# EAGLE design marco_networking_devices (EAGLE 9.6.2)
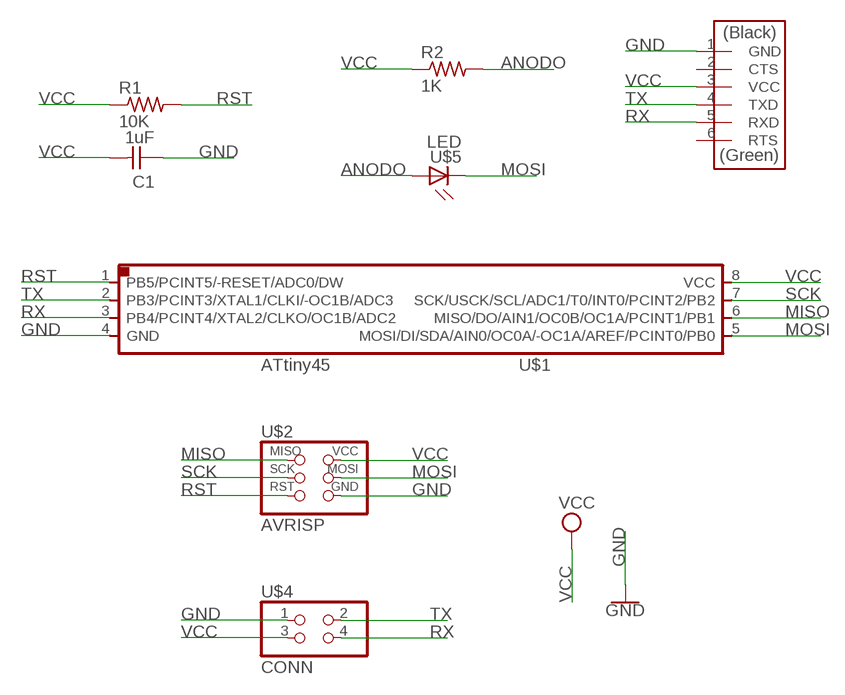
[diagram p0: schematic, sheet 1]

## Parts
C1  1uF  CAP_UNPOLARIZEDFAB  [C1206FAB]
R1  10K  R1206FAB  [R1206FAB]
R2  1K  R1206FAB  [R1206FAB]
U$1  ATTINY45  UC_ATTINY45SI  [SOIC8]
U$2  AVRISP  CONN_03X2_AVRISPSMD  [2X03SMD]
U$3  FTDI  CONN_06_FTDI-SMD-HEADER  [1X06SMD]
U$4  CONN  CONN_02X2-PINHEAD-SMD  [2X02SMD]
U$5  LED  LEDFAB1206  [LED1206FAB]

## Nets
ANODO: R2.2 U$5.1(A)
GND: C1.1 U$1.4(GND) U$2.6(GND) U$3.1(GND) U$4.1
MISO: U$1.6(MISO/DO/AIN1/OC0B/OC1A/PCINT1/PB1) U$2.1(MISO)
MOSI: U$1.5(MOSI/DI/SDA/AIN0/OC0A/-OC1A/AREF/PCINT0/PB0) U$2.4(MOSI) U$5.2(C)
RST: R1.2 U$1.1(PB5/PCINT5/-RESET/ADC0/DW) U$2.5(RST)
RX: U$1.3(PB4/PCINT4/XTAL2/CLKO/OC1B/ADC2) U$3.5(RXD) U$4.4
SCK: U$1.7(SCK/USCK/SCL/ADC1/T0/INT0/PCINT2/PB2) U$2.3(SCK)
TX: U$1.2(PB3/PCINT3/XTAL1/CLKI/-OC1B/ADC3) U$3.4(TXD) U$4.2
VCC: C1.2 R1.1 R2.1 U$1.8(VCC) U$2.2(VCC) U$3.3(VCC) U$4.3
Unconnected: U$3.2(CTS) U$3.6(RTS)

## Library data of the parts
C1 = fab:CAP_UNPOLARIZED
R1 R2 = fab:R: Resistor (US Symbol)
U$1 = fab:UC_ATTINY45
U$2 = fab:CONN_03X2_AVRISP
U$3 = fab:CONN_06_FTDI-SMD-HEADER
U$4 = fab:CONN_02X2-PINHEAD-SMD
U$5 = fab:LED: LED

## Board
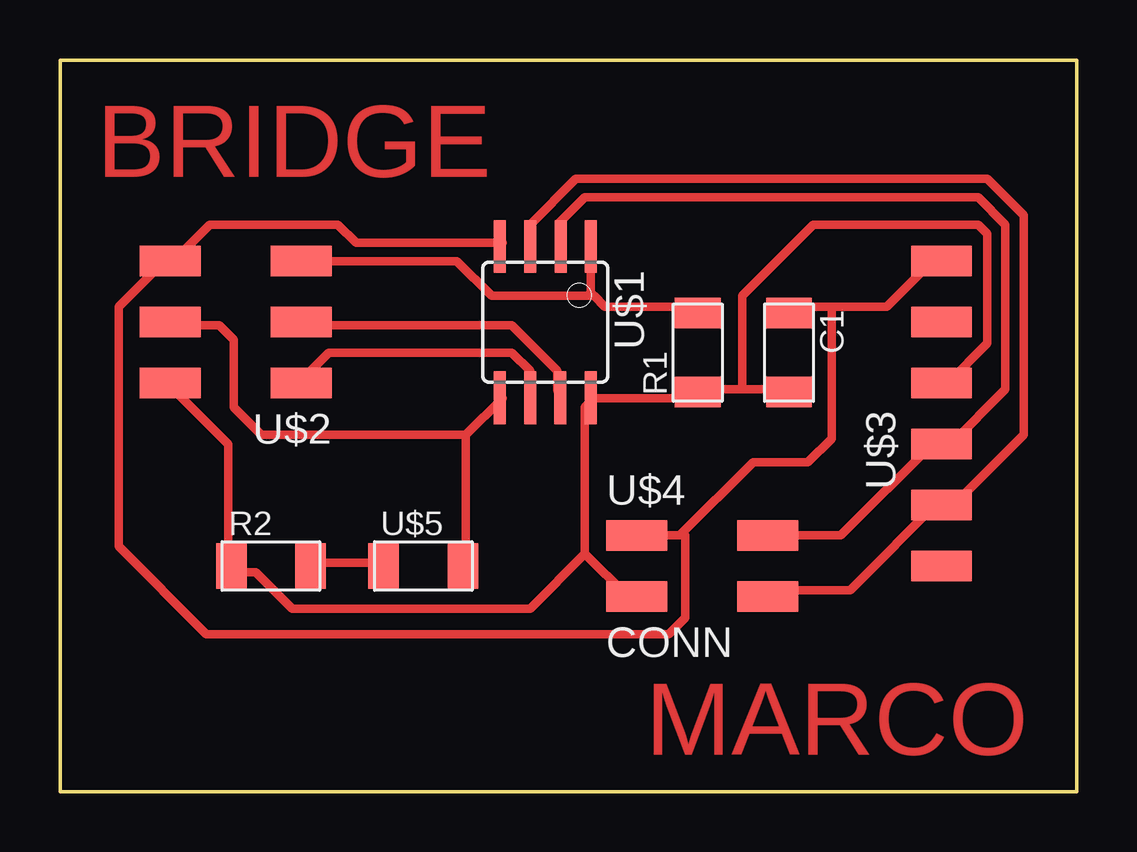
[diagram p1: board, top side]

Size 42.37 x 30.48 mm. Coordinates in mm from the lower left corner, seen from the top.
Outline: 0,30.48 42.37,30.48 42.37,0 0,0 0,30.48
Copper layers (1*16): Top 0.035mm / dielectric 1.5mm / Bottom 0.035mm
Design rules "fabcity-designrules *": minimum track width 14mil, minimum drill 32mil, track to track 16mil, track to pad 16mil, pad to pad 16mil, via to via 16mil, smd to smd 6mil, copper to edge 16mil, drill to drill 16mil, minimum pad ring 10mil, minimum via ring 8mil, stop-mask expansion 4mil, vias tented up to drill 0mil, thermal gap 16mil

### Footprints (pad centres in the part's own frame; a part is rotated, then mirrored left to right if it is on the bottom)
C1206FAB = smd 1.27 x 1.905: 1 -1.651,0; 2 1.651,0
R1206FAB = smd 1.27 x 1.905: 1 -1.651,0; 2 1.651,0
SOIC8 = smd 0.5 x 2.2: 1 -1.905,-3.154; 2 -0.645,-3.154; 3 0.625,-3.154; 4 1.895,-3.154; 5 1.905,3.154; 6 0.635,3.154; 7 -0.635,3.154; 8 -1.905,3.154
2X03SMD = smd 2.54 x 1.27: 1 -2.54,2.54; 2 2.92,2.54; 3 -2.54,0; 4 2.92,0; 5 -2.54,-2.54; 6 2.92,-2.54
1X06SMD = smd 2.54 x 1.27: 1 0,6.35; 2 0,3.81; 3 0,1.27; 4 0,-1.27; 5 0,-3.81; 6 0,-6.35
2X02SMD = smd 2.54 x 1.27: 1 -2.54,1.27; 2 2.92,1.27; 3 -2.54,-1.27; 4 2.92,-1.27
LED1206FAB = smd 1.27 x 1.905: 1 -1.651,0; 2 1.651,0

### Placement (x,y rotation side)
C1  30.38,18.29 270 top
R1  26.57,18.29 90 top
R2  8.79,9.4 0 top
U$1  20.22,19.56 180 top
U$2  7.52,19.56 180 top
U$3  36.73,15.75 0 top
U$4  26.57,9.4 0 top
U$5  15.14,9.4 0 top

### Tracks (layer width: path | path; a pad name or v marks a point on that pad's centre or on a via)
ANODO
  Top 0.356: R2.2 10.44,9.53 13.49,9.53 U$5.1
GND
  Top 0.356: U$1.4 18.44,22.86 12.34,22.86 11.58,23.62 6.25,23.62 4.72,22.1 U$2.6 4.34,22.1 2.44,20.19 2.44,10.21 6.1,6.55 25.37,6.55 26.06,7.24 26.06,10.67 25.83,10.67 | 32.16,20.19 34.44,20.19 36.35,22.1 U$3.1 | 32.16,20.19 30.63,20.19 C1.1 | 25.83,10.67 U$4.1 | 25.83,10.67 28.88,13.72 31.17,13.72 32.16,14.71 32.16,20.19
MISO
  Top 0.356: U$1.6 19.58,17.53 18.82,18.29 11.2,18.29 10.06,17.14 U$2.1
MOSI
  Top 0.356: 16.92,14.86 16.92,9.53 U$5.2 | 16.92,14.86 18.44,16.38 U$1.5 | 16.92,14.86 8.38,14.86 7.24,16 7.24,18.82 6.63,19.43 4.72,19.43 U$2.4
RST
  Top 0.356: 22.25,20.65 22.1,20.8 22.1,20.78 22.12,20.73 U$1.1 | 22.25,20.65 22.71,20.19 26.44,20.19 R1.2 | U$2.5 16.54,22.1 17.98,20.65 22.25,20.65
RX
  Top 0.356: 36.73,12.19 37.49,12.19 40.16,14.86 40.16,24 38.63,25.53 21.49,25.53 19.58,23.62 19.58,22.86 U$1.3 | 36.73,12.19 32.92,8.38 29.49,8.38 U$4.4 | 36.73,12.19 U$3.5
SCK
  Top 0.356: U$1.7 20.73,16.76 20.73,17.53 18.82,19.43 10.06,19.43 U$2.3
TX
  Top 0.356: U$1.2 20.8,22.77 20.8,23.7 21.87,24.77 38.25,24.77 39.4,23.62 39.4,16.76 37.11,14.48 U$3.4 36.35,14.48 32.54,10.67 U$4.2
VCC
  Top 0.356: U$2.2 4.72,16.76 7.01,14.48 7.01,9.53 R2.1 7.39,9.14 8.15,9.14 9.68,7.62 19.58,7.62 21.87,9.91 | 28.42,16.76 30.25,16.76 C1.2 | 28.42,16.76 26.82,16.76 R1.1 26.44,16.38 22.25,16.38 | U$4.3 23.65,8.13 21.87,9.91 | 21.87,9.91 21.87,16 22.25,16.38 | 22.25,16.38 U$1.8 | U$3.3 36.98,17.02 38.63,18.67 38.63,23.24 38.25,23.62 31.39,23.62 28.42,20.65 28.42,16.76

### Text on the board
Top: BRIDGE | MARCO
